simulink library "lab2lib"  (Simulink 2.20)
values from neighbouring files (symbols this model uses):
  a = 1    [init_exercise.m]
  ad = 2*cos(wd)    [init_exercise.m]
  am = 0.5    [init_exercise.m]
  b = 1    [init_exercise.m]
libraries: adaptlib x2

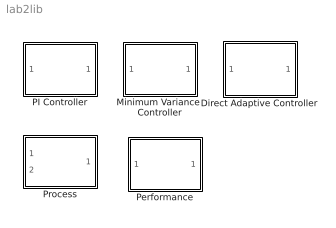
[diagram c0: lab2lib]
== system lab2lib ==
  Direct Adaptive Controller : Subsystem
  Minimum Variance  Controller : Subsystem
  PI Controller : Subsystem
  Performance : Subsystem
  Process : Subsystem

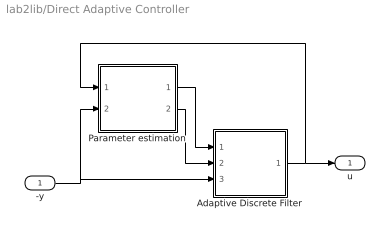
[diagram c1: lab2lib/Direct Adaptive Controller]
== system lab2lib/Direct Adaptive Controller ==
  -y : Inport  Port=1  PortWidth=-1  SampleTime=-1
  Adaptive Discrete Filter : Subsystem  mask{n_N=2, n_D=2, h=1}
      mask prompts: n_N "n_N (degree numerator)"; n_D "n_D (degree denominator)"
  Parameter estimation : Subsystem
  u : Outport  Port=1
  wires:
  -y/1 -> Parameter estimation/2(-y), Adaptive Discrete Filter/3(In3)
  Adaptive Discrete Filter/1(Out1) -> u/1, Parameter estimation/1(u)
  Parameter estimation/2(R) -> Adaptive Discrete Filter/2(In2)
  Parameter estimation/1(S) -> Adaptive Discrete Filter/1(In1)

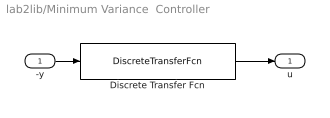
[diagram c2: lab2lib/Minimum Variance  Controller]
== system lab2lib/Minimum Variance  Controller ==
  -y : Inport  Port=1  PortWidth=-1  SampleTime=-1
  Discrete Transfer Fcn : DiscreteTransferFcn  Numerator=[(a+ad)/b -(1+ad)/b a/b]  Denominator=[1 -ad 1]  SampleTime=1
  u : Outport  Port=1  InitialOutput=0
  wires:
  Discrete Transfer Fcn/1 -> u/1
  -y/1 -> Discrete Transfer Fcn/1

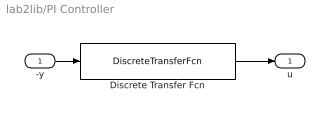
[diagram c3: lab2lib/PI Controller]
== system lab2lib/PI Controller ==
  -y : Inport  Port=1  PortWidth=-1  SampleTime=-1
  Discrete Transfer Fcn : DiscreteTransferFcn  Numerator=[(1+a-am)/b -a/b]  Denominator=[1 -1]  SampleTime=1
  u : Outport  Port=1  InitialOutput=0
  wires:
  Discrete Transfer Fcn/1 -> u/1
  -y/1 -> Discrete Transfer Fcn/1

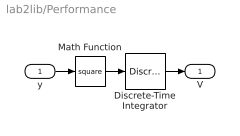
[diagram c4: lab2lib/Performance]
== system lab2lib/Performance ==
  y : Inport  Port=1  PortWidth=-1  SampleTime=-1
  Discrete-Time Integrator : DiscreteIntegrator  IntegratorMethod=ForwardEuler  ExternalReset=none  InitialConditionSource=internal  InitialCondition=0  LimitOutput=off  UpperSaturationLimit=inf  LowerSaturationLimit=-inf  ShowSaturationPort=off  ShowStatePort=off  SampleTime=1
  Math Function : Math  Operator=square
  V : Outport  Port=1
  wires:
  y/1 -> Math Function/1
  Math Function/1 -> Discrete-Time Integrator/1
  Discrete-Time Integrator/1 -> V/1

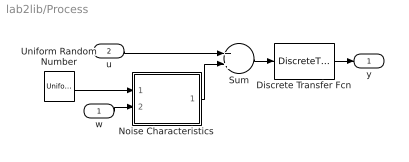
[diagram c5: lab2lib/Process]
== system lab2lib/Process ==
  w : Inport  Port=1  PortWidth=-1  SampleTime=-1
  u : Inport  Port=2  PortWidth=-1  SampleTime=-1
  Discrete Transfer Fcn : DiscreteTransferFcn  Numerator=[b]  Denominator=[1 -a]  SampleTime=1
  Noise Characteristics : Subsystem
  Sum : Sum  Inputs=++
  Uniform Random Number : UniformRandomNumber  Minimum=-0.1  Maximum=0.1  Seed=0  SampleTime=0
  y : Outport  Port=1  InitialOutput=0
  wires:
  Sum/1 -> Discrete Transfer Fcn/1
  u/1 -> Sum/1
  Uniform Random Number/1 -> Noise Characteristics/1(u)
  w/1 -> Noise Characteristics/2(w)
  Discrete Transfer Fcn/1 -> y/1
  Noise Characteristics/1(y) -> Sum/2

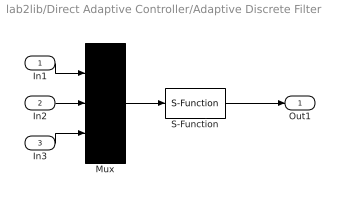
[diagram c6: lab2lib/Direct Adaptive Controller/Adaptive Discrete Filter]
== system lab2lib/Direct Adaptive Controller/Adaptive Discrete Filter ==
  In1 : Inport  Port=1  PortWidth=-1  SampleTime=-1
  In2 : Inport  Port=2  PortWidth=-1  SampleTime=-1
  In3 : Inport  Port=3  PortWidth=-1  SampleTime=-1
  Mux : Mux  Inputs=[n_N+1 n_D+1 1]
  S-Function : S-Function  FunctionName=zfilter  Parameters=n_D,n_N,h  PortCounts=[]  SFunctionModules=''
  Out1 : Outport  Port=1
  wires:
  S-Function/1 -> Out1/1
  Mux/1 -> S-Function/1
  In3/1 -> Mux/3
  In2/1 -> Mux/2
  In1/1 -> Mux/1

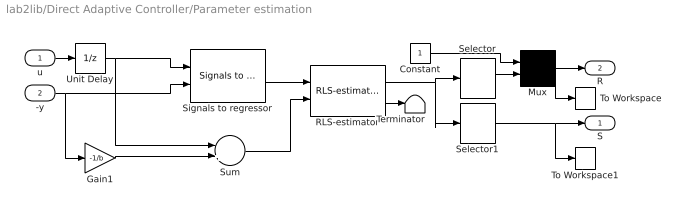
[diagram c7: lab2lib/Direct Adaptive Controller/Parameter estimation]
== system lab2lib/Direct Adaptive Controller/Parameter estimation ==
  u : Inport  Port=1  PortWidth=-1  SampleTime=-1
  -y : Inport  Port=2  PortWidth=-1  SampleTime=-1
  Constant : Constant  Value=1
  Gain1 : Gain  Gain=-1/b
  Mux : Mux  Inputs=2
  RLS-estimator : adaptlib/RLS-estimator  n=5  theta_0=[-1.99; 1; 2.99; -2.99; 1]  P_0=10*eye(5)  lambda=1  h=1
  Selector : Selector  Elements=[1 2]  InputPortWidth=5
  Selector1 : Selector  Elements=[3 4 5]  InputPortWidth=5
  Signals to regressor : adaptlib/Signals to regressor  m=2  n=3  h=1
  Sum : Sum  Inputs=-+
  Terminator : Terminator
  To Workspace : ToWorkspace  VariableName=R  SampleTime=-1
  To Workspace1 : ToWorkspace  VariableName=S  SampleTime=-1
  Unit Delay : UnitDelay  X0=0  SampleTime=1
  S : Outport  Port=1  InitialOutput=0
  R : Outport  Port=2  InitialOutput=0
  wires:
  RLS-estimator/1 -> Selector/1, Selector1/1
  RLS-estimator/2 -> Terminator/1
  Sum/1 -> RLS-estimator/2
  -y/1 -> Gain1/1, Signals to regressor/2
  Selector/1 -> Mux/2
  Constant/1 -> Mux/1
  Signals to regressor/1 -> RLS-estimator/1
  u/1 -> Unit Delay/1
  Unit Delay/1 -> Sum/1, Signals to regressor/1
  Gain1/1 -> Sum/2
  Mux/1 -> R/1, To Workspace/1
  Selector1/1 -> S/1, To Workspace1/1

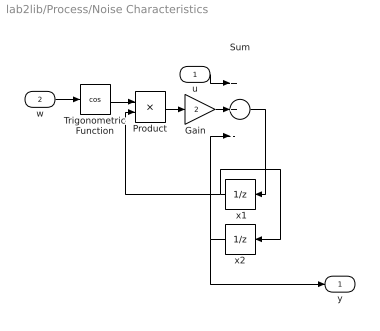
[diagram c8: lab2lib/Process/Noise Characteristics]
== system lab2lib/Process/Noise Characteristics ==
  u : Inport  Port=1  PortWidth=-1  SampleTime=-1
  w : Inport  Port=2  PortWidth=-1  SampleTime=-1
  " x1" : UnitDelay  Orientation=left  X0=0  SampleTime=1
  Gain : Gain  Gain=2
  Product : Product  Inputs=2
  Sum : Sum  Inputs=++-
  Trigonometric Function : Trigonometry  Operator=cos
  x2 : UnitDelay  Orientation=left  X0=0  SampleTime=1
  y : Outport  Port=1  InitialOutput=0
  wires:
  w/1 -> Trigonometric Function/1
  Gain/1 -> Sum/2
  Product/1 -> Gain/1
  Trigonometric Function/1 -> Product/1
  Sum/1 -> " x1"/1
  " x1"/1 -> Product/2, x2/1
  u/1 -> Sum/1
  x2/1 -> Sum/3, y/1
